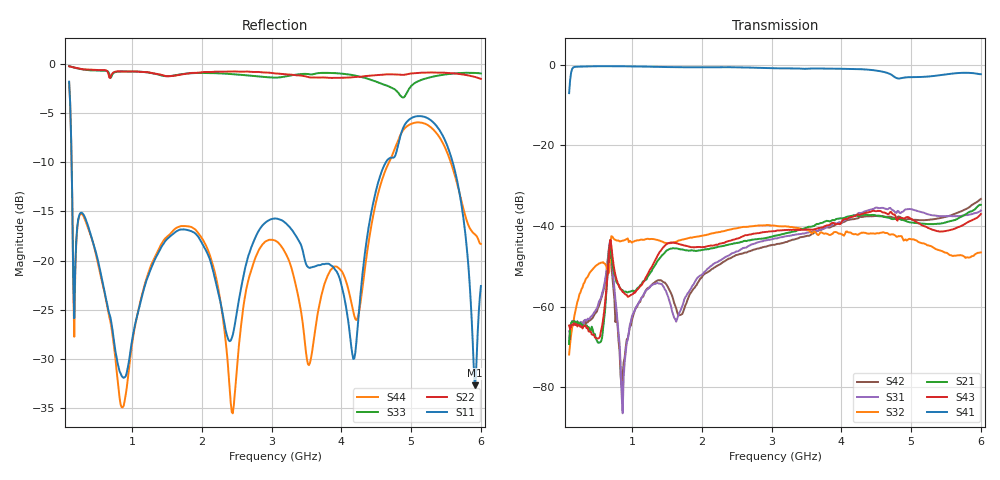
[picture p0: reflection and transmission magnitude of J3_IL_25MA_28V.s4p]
!Keysight Technologies,N5242B,MY61256241,Z.15.82.127
!Date: Friday, August 25, 2023 02:21:39
!Correction: S11(C  4-Port  )
!S12(C  4-Port  )
!S13(C  4-Port  )
!S14(C  4-Port  )
!S21(C  4-Port  )
!S22(C  4-Port  )
!S23(C  4-Port  )
!S24(C  4-Port  )
!S31(C  4-Port  )
!S32(C  4-Port  )
!S33(C  4-Port  )
!S34(C  4-Port  )
!S41(C  4-Port  )
!S42(C  4-Port  )
!S43(C  4-Port  )
!S44(C  4-Port  )
!S4P File: Measurements: <S11,S12,S13,S14>,
!<S21,S22,S23,S24>,
!<S31,S32,S33,S34>,
!<S41,S42,S43,S44>:
# Hz S  dB  R 50
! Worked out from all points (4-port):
!   401 points, 100 MHz to 6 GHz, reference 50 ohm
!   strongest paths, dB at 100 MHz, 1.575 GHz, 3.05 GHz, 4.525 GHz, 6 GHz:
!     S41: -7.0, -0.6, -0.9, -1.5, -2.4
!     S43: -64.7, -44.1, -41.3, -36.2, -37.0
!     S21: -69.3, -45.6, -42.4, -37.4, -34.8
!     S32: -71.9, -44.2, -39.9, -41.8, -46.6
!     S31: -66.1, -61.1, -43.1, -35.5, -36.2
!     S42: -68.7, -57.3, -44.6, -37.6, -33.3
!   lowest |S11| = -32.7 dB at 5.912 GHz (marker M1), VSWR 1.05, Z = 48.3 + j1.54 ohm
!   |S11| at or under -10 dB: 135.4 MHz to 4.639 GHz (4.504 GHz wide, 189 % of centre); 5.596 GHz to end of sweep
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1e8  -1.82 -105.1  -69.83 -96.4  -66.31 160.1  -7.05 154.1
     -69.27 -90.0  -0.26 -72.6  -70.98 -162.8  -68.24 -70.9
     -66.08 159.1  -71.88 -164.9  -0.24 -74.3  -64.80 165.9
     -7.05 154.1  -68.74 -73.8  -64.68 165.0  -1.87 -106.5
5.425e8  -20.93 -155.6  -68.73 -87.5  -58.13 -8.8  -0.37 -78.2
         -68.86 -92.7  -0.64 122.2  -49.22 15.4  -58.87 9.0
         -58.31 -8.3  -49.24 15.4  -0.69 91.5  -67.40 -124.1
         -0.37 -78.2  -58.94 7.6  -67.43 -123.5  -21.23 -151.4
1.44225e9  -18.39 155.6  -47.11 -103.2  -54.81 117.3  -0.57 92.7
           -47.12 -102.8  -1.17 -62.8  -43.90 162.9  -53.85 -157.6
           -54.81 118.2  -43.90 162.6  -1.22 -143.2  -45.48 -130.9
           -0.57 92.7  -53.82 -156.9  -45.43 -131.1  -18.08 -168.3
2.35675e9  -27.48 -76.8  -44.72 76.0  -47.56 45.2  -0.62 -86.3
           -44.74 76.1  -0.80 138.3  -41.12 -12.7  -48.40 97.8
           -47.54 45.3  -41.10 -12.8  -1.01 18.1  -43.88 20.6
           -0.62 -86.2  -48.39 97.9  -43.88 20.5  -29.12 45.6
4.6725e9  -9.69 60.9  -37.93 3.0  -35.79 -126.2  -2.13 171.7
          -37.94 2.9  -1.07 88.8  -41.90 -124.4  -37.69 17.0
          -35.79 -126.1  -41.91 -124.2  -2.27 -163.3  -37.10 -94.7
          -2.12 171.8  -37.72 17.0  -37.12 -94.9  -10.18 94.2
5.9115e9  -32.66 136.7  -35.93 171.1  -36.85 -16.1  -2.14 -64.9
          -35.92 171.2  -1.33 -83.5  -47.14 17.2  -34.39 179.6
          -36.81 -16.0  -47.08 17.3  -0.93 -52.6  -38.25 47.4
          -2.14 -64.8  -34.39 179.7  -38.23 47.6  -17.31 -56.5
6e9  -22.58 29.1  -34.76 152.5  -36.15 -29.5  -2.36 -82.7
     -34.76 152.5  -1.53 -99.3  -46.53 1.1  -33.28 162.6
     -36.15 -29.4  -46.55 0.6  -0.98 -66.3  -37.03 33.9
     -2.36 -82.6  -33.30 162.7  -37.03 33.8  -18.31 -50.3
